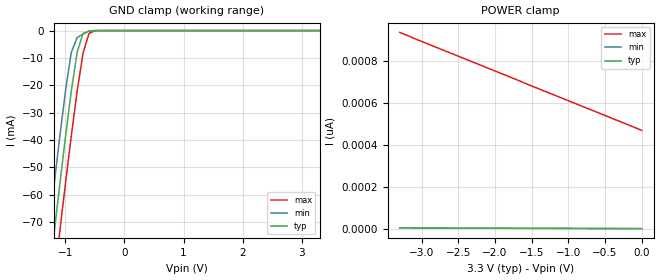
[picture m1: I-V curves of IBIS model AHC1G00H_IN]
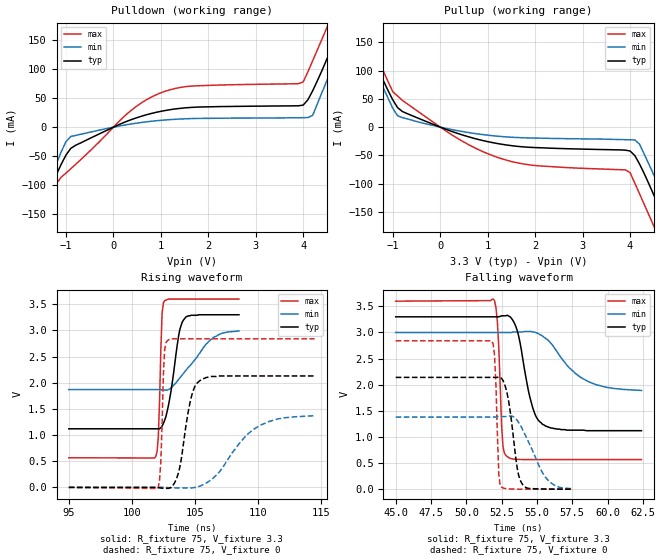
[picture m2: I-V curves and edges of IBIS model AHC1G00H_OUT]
| TEXAS INSTRUMENTS INCORPORATED
| Standard Linear and Logic Group
| IBIS Model of SN74AHC1G00H
| SINGLE 2-INPUT POSITIVE-NAND GATE
| MPAK-5 5-pin (DBV) Package
[IBIS Ver]   2.1
[Comment Char]  |_char
[File name]   ul00_3m.ibs
[File Rev]   2.0
[Date]   April 26, 2000
[Source]   Data created from SPICE simulations at Hitachi,Ltd.
[Notes]   The following is an IBIS List for the AHC1G00H.
|   Please contact sllibis@ti.com with questions and
|   comments concerning SLL IBIS models.
[Disclaimer] Property of Texas Instruments Incorporated.  Unauthorized
   reproduction and/or distribution is strictly prohibited.
   This product is protected under copyright law.
   Created 2000, (C) Copyright 2000, Texas Instruments Inc.,
   All Rights Reserved.
   UNLESS THERE IS A SIGNED, WRITTEN AGREEMENT TO THE
   CONTRARY, TEXAS INSTRUMENTS () IS PROVIDING THE IBIS
   MODELS  AND WITHOUT ANY WARRANTY, EXPRESSED OR
   IMPLIED.  TI assumes no liability for:
   1) the accuracy of the IBIS models provided to your
   company;
   2) the proper functioning of these IBIS Models in your
   design or for any resulting applications; or
   3) infringement of patents, copyrights or intellectual
   property rights resulting from your use of these IBIS
   models.
   TI provides IBIS Models as a service to our customers.
   You and your company shall not distribute, sell or give
   these models to anyone else without prior written
   permission from TI.
   TI reserves the right to make changes to our products or
   to discontinue any semiconductor product or service
   without notice, and advises our customers to obtain the
   latest version of relevant information to verify, before
   placing orders, that the information being relied on is
   current.
   Please be aware that your receipt and use of the IBIS
   information provided shall serve as acceptance of these
   terms and conditions.  If you do not accept these terms,
   you should return or destroy the IBIS models and any
   other accompanying information immediately.
|   Component AHC1G00H
[Component]   AHC1G00H
[Manufacturer]   Hitachi, Ltd.
[Package]
|   typ   min   max
R_pkg   0.089   0.050   0.104
L_pkg   1.520nH   0.920nH   1.720nH
C_pkg   0.240pF   0.150pF   0.520pF
[Pin]   signal_name   model_name   R_pin   L_pin   C_pin
1   A   AHC1G00H_IN   0.097   1.620nH   0.150pF
2   B   AHC1G00H_IN   0.050   0.920nH   0.210pF
3   GND   GND   0.092   1.640nH   0.520pF
4   Y   AHC1G00H_OUT   0.104   1.720nH   0.160pF
5   VCC   POWER   0.103   1.710nH   0.150pF
| Models and submodels in the file (2): AHC1G00H_IN (Input), AHC1G00H_OUT (Output)
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|   Model AHC1G00H_IN
[Model]   AHC1G00H_IN
Model_type  Input
Polarity   Inverting
Vinl = 0.99
Vinh = 2.31
| variable   typ   min   max
C_comp   1.80pF   1.73pF   1.97pF
[Temperature Range]   25   85   -40
[Voltage Range]   3.3   3.0   3.6
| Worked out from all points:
|   GND clamp passes 1 mA (typ) near -0.70 V on its own axis
[GND Clamp]
|   Voltage   I(typ)   I(min)   I(max)
-3.3V     -486mA     -469mA     -503mA
-1.3V     -94.6mA    -76.9mA    -112mA
-1.2V     -75.8mA    -58.1mA    -93.1mA
-1.1V     -57.3mA    -39.8mA    -74.5mA
-1V       -39.2mA    -22.4mA    -56.2mA
-900mV    -22.2mA    -7.98mA    -38.6mA
-800mV    -7.87mA    -2.53mA    -22mA
-700mV    -1.03mA    -1.34mA    -8.2mA
-600mV    -206uA     -154uA     -1.06mA
-500mV    -11.2uA    -2.6uA     -57.2uA
3.3V      3.55pA     3.3pA      469pA
[POWER Clamp]
|   Voltage   I(typ)   I(min)   I(max)
-3.3V     7pA        6.6pA      934pA
-1.6V     5.23pA     4.9pA      694pA
-100mV    3.66pA     3.4pA      484pA
0V        3.55pA     3.3pA      469pA
|   Model AHC1G00H_OUT
[Model]   AHC1G00H_OUT
Model_type  Output
Polarity   Non-Inverting
Vmeas = 1.65
Cref = 15pf
| variable   typ   min   max
C_comp   3.84pF   3.72pF   3.96pF
[Temperature Range]   25   85   -40
[Voltage Range]   3.3   3.0   3.6
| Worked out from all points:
|   slope of the pulldown table from 0 to 0.495 V, typ, clamps not added: 30.4 ohm
|   slope of the pullup table from 0 to 0.495 V, typ, clamps not added: 34 ohm
|   rising waveform, R_fixture 75, V_fixture 3.3: 20-80 % time 794ps typ, 2.21ns min, 222ps max; typ from 1.12 V to 3.3 V
|   falling waveform, R_fixture 75, V_fixture 3.3: 20-80 % time 947ps typ, 2.25ns min, 267ps max; typ from 3.3 V to 1.12 V
|   falling waveform, R_fixture 75, V_fixture 0: 20-80 % time 612ps typ, 1.42ns min, 213ps max; typ from 2.14 V to 0 V
|   rising waveform, R_fixture 75, V_fixture 0: 20-80 % time 856ps typ, 2.72ns min, 217ps max; typ from 0 V to 2.13 V
[Pulldown]
|   Voltage   I(typ)   I(min)   I(max)
-3.3V     -489mA     -473mA     -506mA
-1.8V     -194mA     -179mA     -211mA
-1.6V     -156mA     -142mA     -173mA
-1.2V     -81mA      -62.6mA    -96.6mA
-900mV    -36.6mA    -16.1mA    -71.6mA
1V        27.2mA     11.7mA     59.1mA
3.9V      36.7mA     16.2mA     74.7mA
4.1V      47mA       16.4mA     95.1mA
4.5V      117mA      80.2mA     171mA
4.8V      174mA      137mA      229mA
5V        213mA      175mA      268mA
6.6V      528mA      491mA      584mA
[Pullup]
|   Voltage   I(typ)   I(min)   I(max)
-3.3V     491mA      474mA      508mA
-1.8V     196mA      179mA      214mA
-1.6V     157mA      141mA      175mA
-1V       47.9mA     33.1mA     62.4mA
-900mV    34.5mA     20mA       55.1mA
1.2V      -29mA      -16mA      -53.4mA
3.9V      -40.8mA    -22.2mA    -75.7mA
4.2V      -65.2mA    -30mA      -118mA
4.5V      -120mA     -84.4mA    -175mA
4.8V      -177mA     -138mA     -233mA
5V        -216mA     -177mA     -272mA
6.6V      -533mA     -494mA     -589mA
[Ramp]
| variable   typ   min   max
dV/dt_r   1.28E+00/8.50E-10   8.27E-01/2.76E-09   1.71E+00/2.10E-10
dV/dt_f   1.31E+00/9.40E-10   6.76E-01/2.30E-09   1.82E+00/2.60E-10
R_load = 75
[Rising Waveform]
R_fixture = 75
V_fixture = 3.3
V_fixture_min = 3.0
V_fixture_max = 3.6
|   Time   V(typ)   V(min)   V(max)
95ns      1.12V      1.87V      566mV
101.8ns   1.12V      1.87V      562mV
102.1ns   1.12V      1.87V      960mV
102.4ns   1.17V      1.86V      3.33V
102.6ns   1.28V      1.86V      3.57V
103.1ns   1.83V      1.9V       3.6V
103.8ns   3.01V      2.09V      3.6V
104.1ns   3.2V       2.18V      3.6V
106.5ns   3.3V       2.87V      3.6V
108.5ns   3.3V       2.99V      3.6V
[Falling Waveform]
R_fixture = 75
V_fixture = 3.3
V_fixture_min = 3.0
V_fixture_max = 3.6
|   Time   V(typ)   V(min)   V(max)
45ns      3.3V       3V         3.6V
52ns      3.3V       3V         3.61V
52.2ns    3.3V       3V         3.2V
52.6ns    3.32V      3V         811mV
52.9ns    3.33V      3V         621mV
53.6ns    3.04V      3.01V      570mV
54.5ns    1.76V      3.02V      566mV
55.4ns    1.24V      2.93V      566mV
58.7ns    1.12V      2.05V      566mV
62.4ns    1.12V      1.89V      566mV
[Falling Waveform]
R_fixture = 75
V_fixture = 0
|   Time   V(typ)   V(min)   V(max)
45ns      2.14V      1.38V      2.84V
51.8ns    2.14V      1.38V      2.84V
52ns      2.14V      1.38V      2.56V
52.3ns    2.15V      1.39V      282mV
52.4ns    2.14V      1.39V      65.5mV
52.9ns    1.82V      1.4V       7.74mV
53.6ns    408mV      1.32V      571uV
53.9ns    125mV      1.19V      170uV
55.7ns    2.39mV     197mV      -8uV
57.5ns    207uV      8.38mV     -4uV
[Rising Waveform]
R_fixture = 75
V_fixture = 0
|   Time   V(typ)   V(min)   V(max)
95ns      0V         0V         0V
102ns     -332uV     336uV      -34mV
102.3ns   -12.4mV    754uV      489mV
102.6ns   -17.2mV    -634uV     2.62V
102.9ns   -19.3mV    -5.34mV    2.82V
103.7ns   280mV      -9.68mV    2.84V
104.7ns   1.71V      -10.5mV    2.84V
105.5ns   2.06V      34.3mV     2.84V
110.2ns   2.13V      1.19V      2.84V
114.5ns   2.13V      1.37V      2.84V
